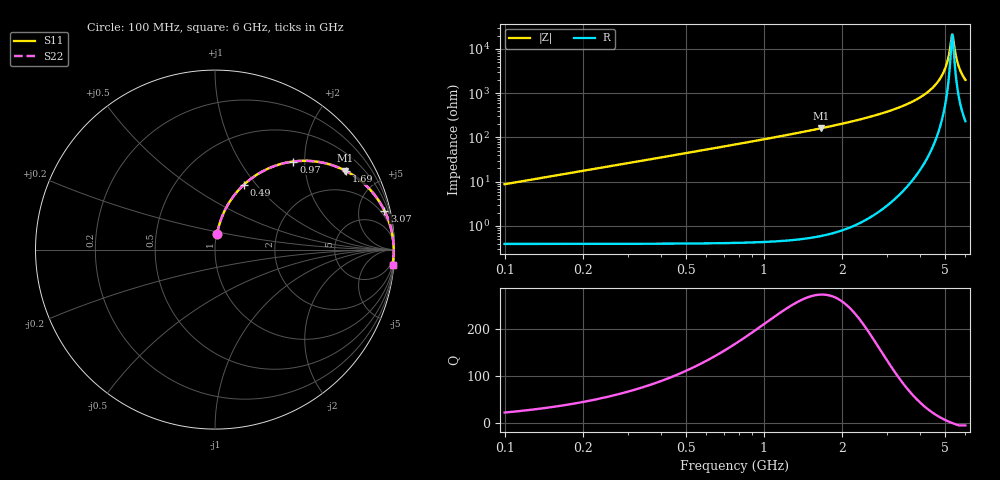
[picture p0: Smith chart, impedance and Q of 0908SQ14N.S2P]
! Coilcraft 0908SQ-14N Air Core Inductor
! 15 June 2010
# MHZ S MA R 50
!Freq  MagS11  AngS11  MagS21  AngS21  MagS12  AngS12  MagS22  AngS22
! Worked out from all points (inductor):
!   395 points, 100 MHz to 6 GHz, reference 50 ohm
!   read as one part in series: L = 13.9 nH near 115 MHz
!   highest Q = 272 at 1.66 GHz (marker M1), where L = 15.4 nH
!   self-resonance near 5.335 GHz
!   S11 on the Smith chart (normalised r, x): 100 MHz: 1.01, +0.17; 490 MHz: 1.01, +0.86; 970 MHz: 1.02, +1.76; 1.69 GHz: 1.05, +3.33; 3.07 GHz: 1.24, +8.64; 6 GHz: 2, -23
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100  0.08674 82.4  0.9923 -5.0  0.9923 -5.0  0.08674 82.4
160  0.138 80.4  0.9866 -8.0  0.9866 -8.0  0.138 80.4
250  0.2129 76.6  0.9733 -12.4  0.9733 -12.4  0.2129 76.6
490  0.3948 66.1  0.9151 -23.4  0.9151 -23.4  0.3948 66.1
970  0.6572 48.3  0.7505 -41.4  0.7505 -41.4  0.6572 48.3
1090  0.703 44.7  0.708 -45.0  0.708 -45.0  0.7031 44.7
1660  0.8473 31.3  0.528 -58.5  0.528 -58.5  0.8473 31.3
1690  0.8524 30.7  0.5197 -59.0  0.5197 -59.0  0.8524 30.7
2080  0.9047 24.3  0.4224 -65.5  0.4224 -65.5  0.9047 24.3
3055  0.9678 13.1  0.2438 -76.5  0.2438 -76.5  0.9679 13.1
3070  0.9684 12.9  0.2416 -76.6  0.2416 -76.6  0.9684 12.9
4045  0.99 5.5  0.1193 -83.2  0.1193 -83.2  0.99 5.5
4645  0.9946 1.8  0.05974 -84.7  0.05974 -84.7  0.9946 1.8
4855  0.9952 0.7  0.04092 -83.8  0.04092 -83.8  0.9953 0.7
5020  0.9955 -0.2  0.02681 -81.3  0.02681 -81.3  0.9955 -0.2
5170  0.9955 -1.0  0.01463 -73.6  0.01463 -73.6  0.9956 -1.0
5320  0.9954 -1.7  0.004953 -23.3  0.004953 -23.3  0.9954 -1.7
5350  0.9953 -1.9  0.00469 5.1  0.00469 5.1  0.9954 -1.9
5485  0.995 -2.5  0.01216 63.8  0.01216 63.8  0.9951 -2.5
5590  0.9947 -3.0  0.01983 72.2  0.01983 72.2  0.9948 -3.0
5770  0.9941 -3.9  0.03304 76.8  0.03304 76.8  0.9941 -3.9
6000  0.993 -4.9  0.04948 78.4  0.04948 78.4  0.9931 -4.9
